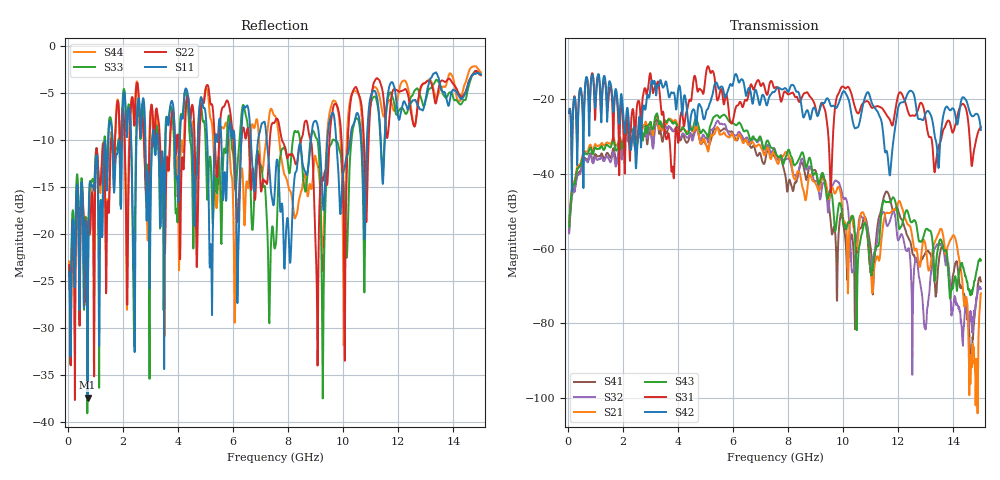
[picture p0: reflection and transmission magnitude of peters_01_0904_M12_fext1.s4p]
# MHZ S RI R 50.00
! FREQ  S11  S12  S13  S14
!  S21  S22  S23  S24
!  S31  S32  S33  S34
!  S41  S42  S43  S44
!  REAL  IMAG  REAL  IMAG  REAL  IMAG  REAL  IMAG
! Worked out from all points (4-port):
!   1496 points, 50 MHz to 15 GHz, reference 50 ohm
!   strongest paths, dB at 50 MHz, 3.79 GHz, 7.53 GHz, 11.27 GHz, 15 GHz:
!     S42: -23.8, -18.4, -17.9, -23.7, -28.3
!     S31: -23.8, -38.7, -17.0, -22.0, -27.6
!     S43: -54.2, -26.4, -34.1, -59.3, -63.2
!     S21: -53.6, -25.8, -35.2, -62.4, -72.0
!     S32: -55.9, -28.5, -33.7, -55.1, -70.7
!     S41: -55.7, -28.4, -35.8, -52.6, -68.8
!   lowest |S11| = -37.4 dB at 720 MHz (marker M1), VSWR 1.03, Z = 49.2 + j1.05 ohm
!   |S11| at or under -10 dB: start of sweep to 1.474 GHz; 7.222 GHz to 8.831 GHz (1.609 GHz wide, 20 % of centre); 9.747 GHz to 10.25 GHz (505.2 MHz wide, 5.05 % of centre)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
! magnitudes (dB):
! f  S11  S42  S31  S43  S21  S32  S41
! 50 MHz  -24.1  -23.8  -23.8  -54.2  -53.6  -55.9  -55.7
! 720 MHz  -37.4  -15.8  -15.3  -34.8  -34.0  -37.0  -36.5
! 3.25 GHz  -9.3  -16.5  -15.8  -24.0  -25.0  -26.4  -25.6
! 3.81 GHz  -6.1  -18.5  -38.1  -26.6  -25.9  -28.6  -28.6
! 5.46 GHz  -9.4  -16.8  -20.2  -24.5  -28.1  -25.9  -27.8
! 10.52 GHz  -7.2  -27.7  -23.8  -66.8  -59.3  -56.3  -55.9
! 15 GHz  -3.1  -28.3  -27.6  -63.2  -72.0  -70.7  -68.8
